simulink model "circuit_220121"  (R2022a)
settings: Solver=VariableStepAuto  StartTime=-D+0.1e-6  StopTime=34e-6  FixedStep=1e-3  MaxStep=0.1e-6  RelTol=1e-3
model workspace (MATLAB code in the model file):
  sGeo = CreateGeometry()
  sConst = CreateConstants()
libraries: fl_lib x8, nesl_utility x3, ee_lib x1

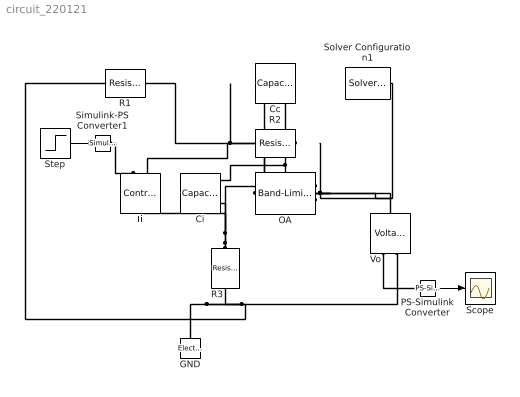
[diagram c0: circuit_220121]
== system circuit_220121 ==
  Cc : fl_lib/Electrical/Electrical Elements/Capacitor  c=0.25 pF  r=0 Ohm  g=0 1/Ohm  i_specify=off  i_priority=None  i=0 A  i_nominal_specify=off  i_nominal_unit=A  i_nominal_value=1  v_specify=off  v_priority=None  v=0 V  v_nominal_specify=off  v_nominal_unit=V  v_nominal_value=1  vc_specify=off  vc_priority=High  vc=0 V  vc_nominal_specify=off  vc_nominal_unit=V  vc_nominal_value=1
  Ci : fl_lib/Electrical/Electrical Elements/Capacitor  c=2 pF  r=0 Ohm  g=0 1/Ohm  i_specify=off  i_priority=None  i=0 A  i_nominal_specify=off  i_nominal_unit=A  i_nominal_value=1  v_specify=off  v_priority=None  v=0 V  v_nominal_specify=off  v_nominal_unit=V  v_nominal_value=1  vc_specify=off  vc_priority=High  vc=0 V  vc_nominal_specify=off  vc_nominal_unit=V  vc_nominal_value=1
  GND : fl_lib/Electrical/Electrical Elements/Electrical Reference
  Ii : fl_lib/Electrical/Electrical Sources/Controlled Current Source
  OA : ee_lib/Integrated Circuits/Band-Limited Op-Amp  A=40000  Rin=1e8 Ohm  Rout=0 Ohm  Vmin=-15 V  Vmax=15 V  Vdotmax=1000000 V/s  f=50 Hz  V0=0 V
  PS-Simulink Converter : nesl_utility/PS-Simulink Converter  PhysicalDomain=network_engine_domain  SubClassName=ps_output  LeftPortType=input  RightPortType=output  PseudoPeriodic=off  Frequencies=[]  VectorFormat=1-D array  Unit=inherit  AffineConversion=off
  R1 : fl_lib/Electrical/Electrical Elements/Resistor  R=1.3 MOhm  i_specify=off  i_priority=None  i=0 A  i_nominal_specify=off  i_nominal_unit=A  i_nominal_value=1  v_specify=off  v_priority=None  v=0 V  v_nominal_specify=off  v_nominal_unit=V  v_nominal_value=1
  R2 : fl_lib/Electrical/Electrical Elements/Resistor  R=5.6 MOhm  i_specify=off  i_priority=None  i=0 A  i_nominal_specify=off  i_nominal_unit=A  i_nominal_value=1  v_specify=off  v_priority=None  v=0 V  v_nominal_specify=off  v_nominal_unit=V  v_nominal_value=1
  R3 : fl_lib/Electrical/Electrical Elements/Resistor  R=1.3 MOhm  i_specify=off  i_priority=None  i=0 A  i_nominal_specify=off  i_nominal_unit=A  i_nominal_value=1  v_specify=off  v_priority=None  v=0 V  v_nominal_specify=off  v_nominal_unit=V  v_nominal_value=1
  Scope : Scope
  Simulink-PS Converter1 : nesl_utility/Simulink-PS Converter  PhysicalDomain=network_engine_domain  SubClassName=ps_input  LeftPortType=input  RightPortType=output  PseudoPeriodic=off  Frequencies=[]  NoiseDistribution=none  NoiseParameters=[]  Unit=1  AffineConversion=off  FilteringAndDerivatives=provide  SimscapeFilterOrder=1  InputFilterTimeConstant=0.001  UdotUserProvided=0
  Solver Configuration1 : nesl_utility/Solver Configuration  PhysicalDomain=network_engine_domain  SubClassName=solver  LeftPortType=input  RightPortType=generic  Tones=[]  Harmonics=[]  SimulateNoise=off  Profile=off  UseLocalSampling=off  EnableSwitchedLinearOptims=on  FrequencyDomain=off  UseCCode=off  RelTol=0.001  AbsTol=1e-06  MinStep=1e-09  ToWorkspace=off  RevertToSquareIcSolve=off  NumHomotopyIterations=100  PhasorMode=off  PhasorModeNumHarmonics=1  IndexReductionMethod=DerivativeReplacement  DoDC=off  ResidualTolerance=1e-09  UseLocalSolver=off  LocalSolverChoice=NE_BACKWARD_EULER_ADVANCER  LocalSolverSampleTime=0.001  DoFixedCost=off  MaxNonlinIter=3  MaxModeIter=2  ComputeImpulses=off  ImpulseIterations=2  LinearAlgebra=Sparse  LinearAlgebraNumThread=0  EquationFormulation=NE_TIME_EF  DelaysMemoryBudget=1024  AutomaticFiltering=on  FilteringTimeConstant=0.001  PartitionStorageMethod=AS_NEEDED  PartitionMemoryBudget=1024  PartitionMethod=FAST
  Step : Step  SampleTime=0
  Vo : fl_lib/Electrical/Electrical Sensors/Voltage Sensor
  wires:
  Step/1 -> Simulink-PS Converter1/1
  PS-Simulink Converter/1 -> Scope/1
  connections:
  R3/RConn1 -- Ii/LConn1 -- OA/LConn1 -- Ci/RConn1
  Vo/RConn1 -- PS-Simulink Converter/LConn1
  OA/RConn1 -- Cc/LConn1 -- R2/LConn1 -- Solver Configuration1/RConn1 -- Vo/LConn1
  Vo/RConn2 -- R3/LConn1 -- R1/RConn1 -- GND/LConn1
  R2/RConn1 -- R1/LConn1 -- Cc/RConn1 -- Ii/RConn2 -- OA/LConn2 -- Ci/LConn1
  Simulink-PS Converter1/RConn1 -- Ii/RConn1
